PROGRAM MAIN
VAR
	bUserEnableAxes:		BOOL	:= TRUE;		(*触发使能功能块，由于是模拟程序，所以直接对轴租进行使能*)
	fUserOverride:			LREAL	:= 100.0;		(*设置通道速比为100%*)
	
	io_X:					AXIS_REF;				(*定义各NC轴*)
	io_Y:					AXIS_REF;
	io_Z:					AXIS_REF;
	io_Q1:					AXIS_REF;
	io_Q2:					AXIS_REF;
	io_Q3:					AXIS_REF;
	
	in_stItpToPlc	AT %I*:	NcToPlc_NciChannel_Ref;	(*定义NCI通道反馈给PLC的一系列状态字等*)
	out_stPlcToItp	AT %Q*:	PLCTONC_NCICHANNEL_REF; (*定义PLC发送给NCI通道的一系列状控制字等*)

	fbEnableAxes:			FB_EnableAxes;			(*调用轴组使能功能块*)
	bAllAxesReady:			BOOL;					(*该变量用于标明轴组使能成功*)
	
	
	fbSimpleNciSequence:	FB_SimpleNciSequence;	(*调用生成NCI通道及执行G代码的功能块*)
	bExecSimpleNci:			BOOL	:= FALSE;		(*用于触发生成NCI通道及执行G代码的功能块*)
	bExeConfirmHsk: 		BOOL	:= FALSE;		(*用于确认M握手指令*)
	sPrgName:				STRING(255) :='Gtest.nc';	(*放置在安装盘中TwinCAT\MC\NCI的文件夹*)
END_VAR

//==========================================
// NciSimpleSample V1.1
//==========================================

//==========================================
// This sample should illustrate how to start up an NCI project.
// Error handling is missing and the sample is not commplete to run a machine.
// 
// To run program copy G-Code file (first.nc) 
// to folder 'C:\TwinCAT\Mc\Nci'.
// Then set bExecSimpleNci to TRUE.
//==========================================
fbEnableAxes(
	bEnableAxes:= bUserEnableAxes, 
	stX:=io_X , 
	stY:=io_Y , 
	stZ:=io_Z , 
	stM1:=io_Q1 , 
	stM2:=io_Q2 , 
	stM3:=io_Q3 , 
	bAllAxesReady=>bAllAxesReady );
	
ItpSetOverridePercent(fOverridePercent:=fUserOverride , sPlcToNci:=out_stPlcToItp);

fbSimpleNciSequence(
	bExecute:=bExecSimpleNci , 
	bConfirmHsk:=bExeConfirmHsk , 
	sPrgName:=sPrgName , 
	bBusy=> , 
	bError=> , 
	bDone=> , 
	stX:=io_X , 
	stY:= io_Y, 
	stZ:= io_Z, 
	st_Q1:=io_Q1 , 
	st_Q2:=io_Q2 , 
	st_Q3:= io_Q3, 
	stItpToPlc:=in_stItpToPlc, 
	stPlcToItp:= out_stPlcToItp);

END_PROGRAM
